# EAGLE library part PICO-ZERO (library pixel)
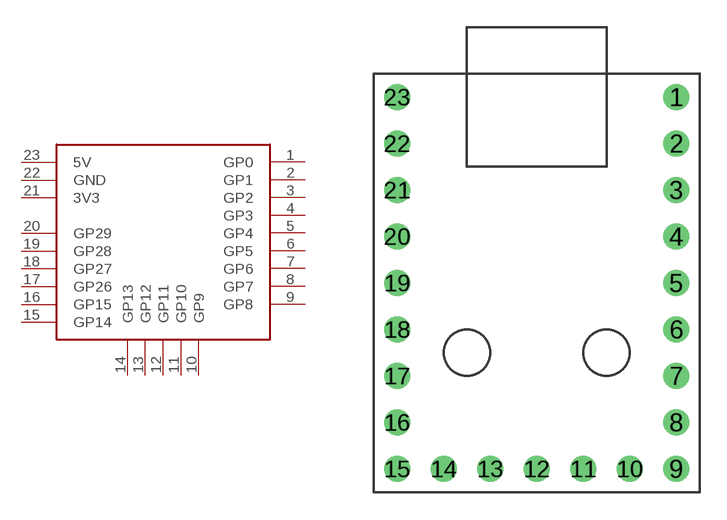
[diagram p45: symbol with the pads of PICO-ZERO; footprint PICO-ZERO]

Designator prefix -

## PICO-ZERO  [PICO-ZERO]
1  GP0
2  GP1
3  GP2
4  GP3
5  GP4
6  GP5
7  GP6
8  GP7
9  GP8
10  GP9
11  GP10
12  GP11
13  GP12
14  GP13
15  GP14
16  GP15
17  GP26
18  GP27
19  GP28
20  GP29
21  3V3
22  GND
23  5V

## Footprint PICO-ZERO (pad centres in mm)
drill 0.9 pad 1.27: 1 7.62,10.16; 2 7.62,7.62; 3 7.62,5.08; 4 7.62,2.54; 5 7.62,0; 6 7.62,-2.54; 7 7.62,-5.08; 8 7.62,-7.62; 9 7.62,-10.16; 10 5.08,-10.16; 11 2.54,-10.16; 12 0,-10.16; 13 -2.54,-10.16; 14 -5.08,-10.16; 15 -7.62,-10.16; 16 -7.62,-7.62; 17 -7.62,-5.08; 18 -7.62,-2.54; 19 -7.62,0; 20 -7.62,2.54; 21 -7.62,5.08; 22 -7.62,7.62; 23 -7.62,10.16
